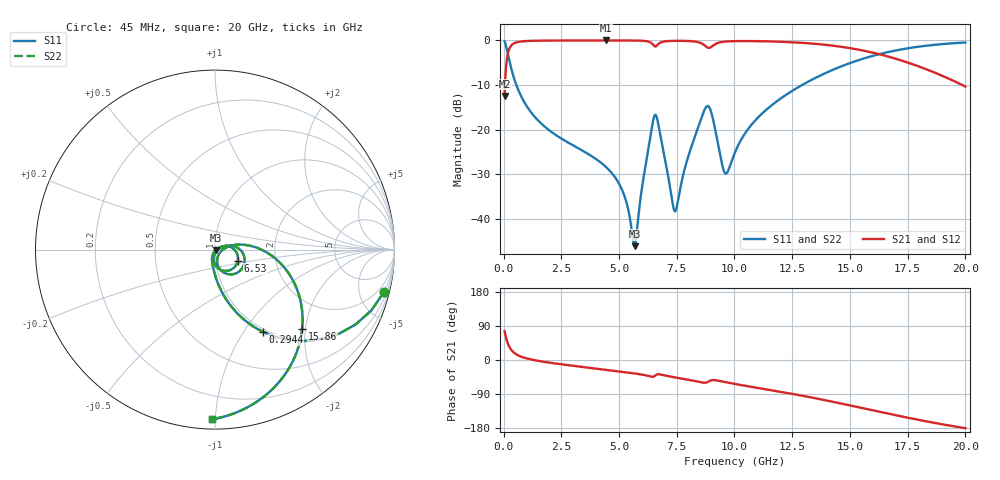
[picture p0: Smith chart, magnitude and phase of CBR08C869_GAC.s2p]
! S-parameter model data by Modelithics Inc.  support@modelithics.com 813-866-6335  Tampa FL USA
! S-Parameter data specifications:
! Substrate: 20-mil Rogers 4350B, substrate thickness, H=0.508mm, Dielectric constant, Er=3.75
! PCB Mounting Pad Footprint: Pad width, PadW=1.45mm , Pad length, PadL=1mm , Pad gap, PadG (edge-to-edge)=0.6mm , Reference planes=2.6mm apart
#  GHz  S  MA  R 50
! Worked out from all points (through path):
!   801 points, 45 MHz to 20 GHz, reference 50 ohm
!   highest |S21| = -0.03 dB at 4.435 GHz (marker M1); lowest = -12.4 dB at 45 MHz (marker M2)
!   group delay of S21, straight-line fit = 26.6 ps
!   lowest |S11| = -46.1 dB at 5.682 GHz (marker M3), VSWR 1.01, Z = 50.4 - j0.304 ohm
!   |S11| at or under -10 dB: 552.8 MHz to 12.93 GHz (12.38 GHz wide, 184 % of centre)
!   |S22| runs from -46.1 to -0.3 dB; largest |S21 - S12| = 0
!   S11 on the Smith chart (normalised r, x): 45 MHz: 0.96, -7.98; 294.4 MHz: 0.96, -1.22; 6.53 GHz: 1.28, -0.17; 15.86 GHz: 1.25, -1.92; 20 GHz: 0.06, -0.98
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0.045  0.9711 -14.1  0.2386 75.9  0.2386 75.9  0.9711 -14.1
0.294438  0.5287 -59.9  0.8483 30.0  0.8483 30.0  0.5287 -59.9
0.593762  0.2966 -76.4  0.9543 13.5  0.9543 13.5  0.2966 -76.4
1.292188  0.1447 -89.6  0.9884 0.1  0.9884 0.1  0.1447 -89.6
3.387462  0.05867 -106.6  0.9964 -18.0  0.9964 -18.0  0.05867 -106.6
4.4351  0.03812 -112.8  0.9968 -25.7  0.9968 -25.7  0.03812 -112.8
5.158469  0.02037 -113.3  0.9964 -31.1  0.9964 -31.1  0.02037 -113.3
5.682288  0.004943 -37.6  0.9944 -35.4  0.9944 -35.4  0.004943 -37.6
6.081387  0.03107 26.0  0.986 -39.5  0.986 -39.5  0.03107 26.0
6.530375  0.1422 -26.5  0.8619 -42.8  0.8619 -42.8  0.1422 -26.5
6.704981  0.1136 -76.4  0.9084 -37.4  0.9084 -37.4  0.1136 -76.4
7.42835  0.01211 -39.7  0.9871 -45.8  0.9871 -45.8  0.01211 -39.7
8.002056  0.05042 20.3  0.9825 -51.8  0.9825 -51.8  0.05042 20.3
8.775313  0.1794 -23.7  0.8481 -59.5  0.8481 -59.5  0.1794 -23.7
8.999806  0.1543 -62.2  0.8463 -53.4  0.8463 -53.4  0.1543 -62.2
9.573512  0.0329 -46.2  0.9668 -58.3  0.9668 -58.3  0.0329 -46.2
10.0225  0.05553 7.8  0.9797 -63.4  0.9797 -63.4  0.05553 7.8
11.16991  0.1492 10.8  0.9771 -75.1  0.9771 -75.1  0.1492 10.8
13.36496  0.3637 -10.9  0.9198 -99.3  0.9198 -99.3  0.3637 -10.9
15.85934  0.6554 -42.2  0.7407 -131.1  0.7407 -131.1  0.6554 -42.2
16.68248  0.7416 -52.9  0.6551 -141.9  0.6551 -141.9  0.7416 -52.9
20  0.9454 -91.0  0.3037 -179.9  0.3037 -179.9  0.9454 -91.0
